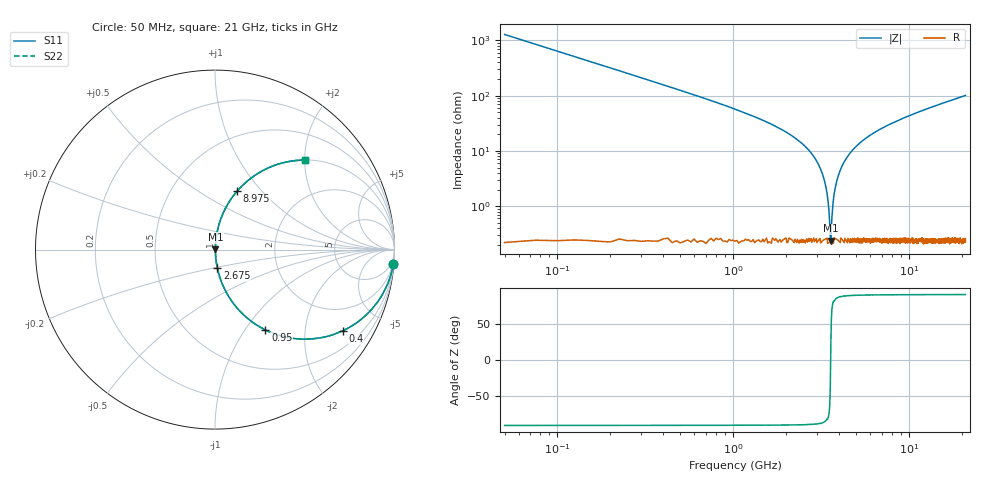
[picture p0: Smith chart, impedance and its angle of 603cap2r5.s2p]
! AVX Thin Film Operation		Date: November 2004
! Description: Accu-P® Series, Thin Film, SMD, RF Capacitor
! Part Number: 06035J2R5ABT
! 50 MHz  -  10.05 GHz
! Serial Measurements
# MHZ S MA R 50
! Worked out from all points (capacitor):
!   839 points, 50 MHz to 21 GHz, reference 50 ohm
!   read as one part in series: C = 2.5 pF near 150 MHz
!   lowest |Z| = 239 mohm at 3.6 GHz (marker M1)
!   series resonance near 3.591 GHz, so ESL is about 790 pH
!   S11 on the Smith chart (normalised r, x): 50 MHz: 1, -25; 400 MHz: 1.01, -3.14; 950 MHz: 1.00, -1.25; 2.675 GHz: 1.00, -0.21; 8.975 GHz: 1.00, +0.74; 21 GHz: 1.00, +2.01
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50  0.997 -4.5  0.078 85.5  0.078 85.5  0.997 -4.5
225  0.942 -19.5  0.334 70.4  0.334 70.4  0.942 -19.5
400  0.843 -32.4  0.536 57.5  0.536 57.5  0.843 -32.4
950  0.528 -57.9  0.847 31.9  0.847 31.9  0.528 -57.9
1600  0.303 -71.9  0.951 17.6  0.951 17.6  0.303 -71.9
2675  0.105 -82.7  0.992 6.0  0.992 6.0  0.105 -82.7
3000  0.064 -84.2  0.996 3.7  0.996 3.7  0.064 -84.2
3250  0.035 -84.1  0.997 2.0  0.997 2.0  0.035 -84.1
3400  0.019 -81.8  0.997 1.1  0.997 1.1  0.019 -81.8
3550  0.004696 -59.0  0.998 0.2  0.998 0.2  0.004696 -59.0
3600  0.002566 20.7  0.998 -0.1  0.998 -0.1  0.002566 20.7
3675  0.008548 73.2  0.998 -0.5  0.998 -0.5  0.008548 73.2
3800  0.02 82.0  0.997 -1.1  0.997 -1.1  0.02 82.0
3925  0.032 83.8  0.997 -1.8  0.997 -1.8  0.032 83.8
4425  0.074 83.9  0.995 -4.3  0.995 -4.3  0.074 83.9
5400  0.147 80.6  0.987 -8.4  0.987 -8.4  0.147 80.6
7050  0.249 75.0  0.966 -14.4  0.966 -14.4  0.249 75.0
8975  0.348 69.3  0.935 -20.4  0.935 -20.4  0.348 69.3
10525  0.416 65.1  0.907 -24.6  0.907 -24.6  0.416 65.1
14025  0.542 56.9  0.838 -32.8  0.838 -32.8  0.542 56.9
17525  0.637 50.2  0.769 -39.6  0.769 -39.6  0.637 50.2
21000  0.709 44.7  0.704 -45.1  0.704 -45.1  0.709 44.7
